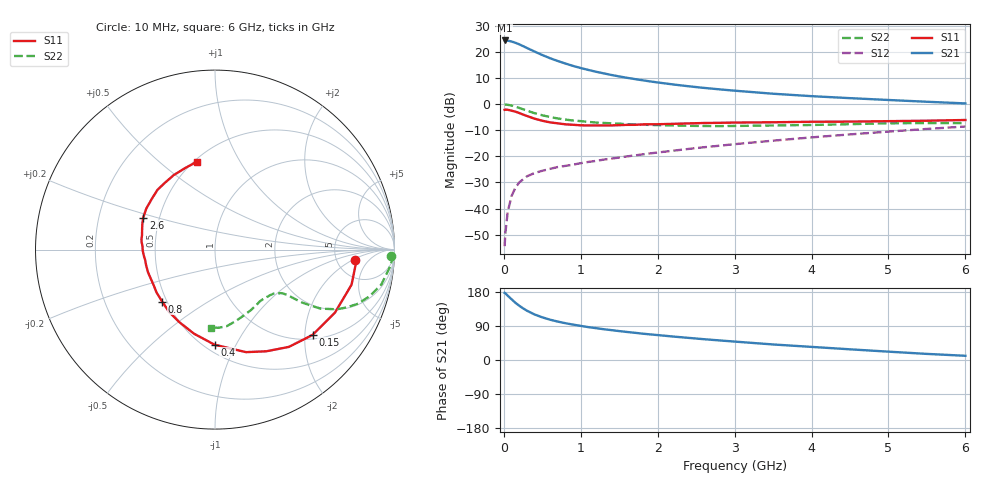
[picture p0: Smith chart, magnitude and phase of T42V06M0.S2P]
! Infineon Technologies  Discrete & RF Semiconductors
! BFR182T
! Si NPN RF Bipolar Junction Transistor in SC75
! VCE = 2 V  IC = 6 mA
! Common Emitter S-Parameters:  October  1999
# GHz  S  MA  R  50
!  f  S11  S21  S12  S22
! GHz  MAG  ANG  MAG  ANG  MAG  ANG  MAG  ANG
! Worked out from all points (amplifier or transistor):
!   36 points, 10 MHz to 6 GHz, reference 50 ohm
!   highest |S21| = 24.5 dB at 10 MHz (marker M1)
!   |S21| within 3 dB of that: start of sweep to 308.4 MHz
!   unconditionally stable (mu >= 1): 1.24 GHz to 3.961 GHz
!   at 250 MHz: K = 0.33, MSG = 25.6 dB, |S12| = -28.8 dB
!   at 1.4 GHz: K = 1.04, MAG = 14.8 dB, |S12| = -20.8 dB
!   at 6 GHz: K = 0.84, MSG = 4.4 dB, |S12| = -8.5 dB
!   lowest NFmin = 1.25 dB at 450 MHz
!   S11 on the Smith chart (normalised r, x): 10 MHz: 7.60, -2.21; 150 MHz: 1.10, -2.19; 400 MHz: 0.56, -0.82; 800 MHz: 0.47, -0.33; 2.6 GHz: 0.41, +0.18; 6 GHz: 0.52, +0.67
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0.01  0.7837 -4.1  16.76 177.2  0.0019 82.6  0.9817 -2.0
0.02  0.7905 -4.5  16.65 176.1  0.0034 95.7  0.9931 -2.5
0.05  0.7856 -14.4  16.64 169.8  0.0086 84.7  0.9765 -6.1
0.1  0.755 -27.7  15.99 160.3  0.0173 77.3  0.9474 -11.8
0.15  0.7221 -41.2  15.14 151.1  0.0251 70.6  0.9008 -16.7
0.2  0.6805 -52.8  14.14 143.2  0.0317 66.8  0.8525 -20.7
0.25  0.6347 -63.2  13.05 136.3  0.0363 61.5  0.8013 -23.7
0.3  0.5968 -73.2  12.02 130.1  0.0415 60.3  0.756 -26.1
0.4  0.5297 -90.3  10.26 120.1  0.0481 55.9  0.674 -29.2
0.5  0.4829 -104.0  8.805 112.6  0.0531 54.0  0.6152 -30.4
0.6  0.4506 -116.1  7.653 106.4  0.0577 53.1  0.5704 -31.2
0.7  0.4311 -126.6  6.771 101.4  0.0626 53.3  0.5351 -31.6
0.8  0.4128 -135.4  6.049 97.1  0.0658 53.7  0.5094 -31.8
1.1  0.3926 -156.8  4.555 86.7  0.0784 55.9  0.4592 -32.6
1.4  0.3933 -171.3  3.647 78.8  0.0908 58.2  0.4321 -34.3
1.6  0.403 -179.3  3.221 74.0  0.1002 59.1  0.4163 -35.5
2.2  0.4218 164.3  2.402 61.9  0.1287 61.7  0.393 -41.8
2.6  0.4375 156.0  2.064 54.9  0.15 62.5  0.3836 -46.8
3.5  0.4518 141.0  1.594 41.0  0.2007 61.9  0.3919 -59.2
4.5  0.4652 126.8  1.311 28.2  0.2646 58.6  0.4155 -74.2
5.5  0.4841 109.9  1.118 16.1  0.3368 53.6  0.4361 -87.6
6  0.4998 101.6  1.039 11.1  0.3747 50.1  0.4348 -93.2
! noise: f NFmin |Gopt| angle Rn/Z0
0.45  1.25  0.25  39  0.3
0.9  1.4  0.25  78  0.23
1.8  1.95  0.21  151  0.2
